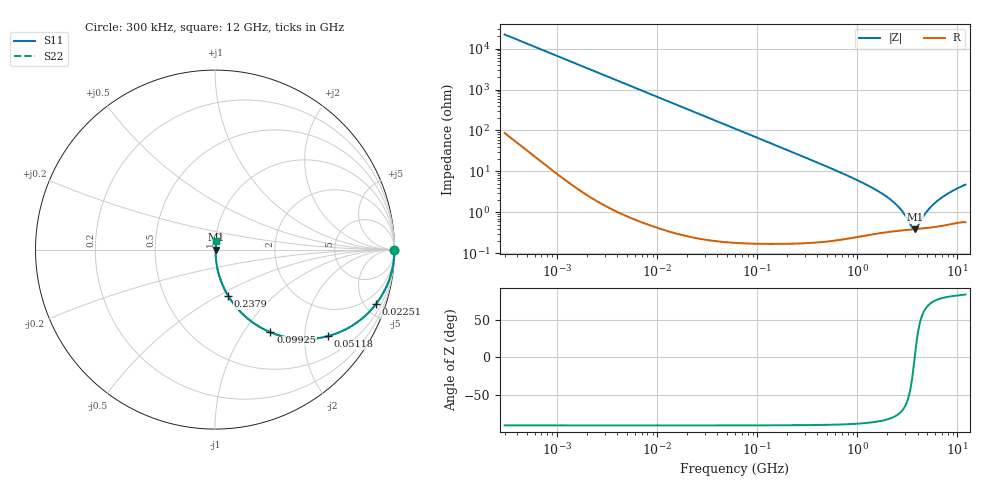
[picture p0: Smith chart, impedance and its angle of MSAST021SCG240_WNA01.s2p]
! MSAST021SCG240_WNA01  S-PARAMETER MODEL  ( Standard Model )
! Model Generated by TAIYO YUDEN Corporation (http://www.ty-top.com)
! Version 1.0
! TAIYO YUDEN Control No. 241126
! Copyright(c) 2024 TAIYO YUDEN CO.,LTD. All Rights Reserved.
! Product Description (link to TY-COMPAS)
! https://ds.yuden.co.jp/TYCOMPAS/or/detail?pn=MSAST021SCG240JWNA01&u=M
! Products Name : Multilayer Ceramic Capacitors
! Characteristics :
!  Capacitance : 24 [pF] , Rated Voltage : 25 [V] , TCC : CG / C0G
!  Case Size : 0.25 x 0.125 / 0.0098 x 0.0049 [mm/inch] , Thickness : 0.125 / 0.0049 [mm/inch]
!  (Conditions: Temperature = 25 [degC] , DC Bias Voltage = 0 [V])
! External Node Assignments :
!  1  o---| |---o  2
! GND o---------o GND
! Frequency Range : 0.3MHz  -  12000MHz  [ 401 STEP ]
# MHZ S RI R 50
! Freq[MHz].  S11 Real  S11 Imag  S21 Real  S21 Imag  S12 Real  S12 Imag  S22 Real  S22 Imag
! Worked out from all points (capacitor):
!   401 points, 300 kHz to 12 GHz, reference 50 ohm
!   read as one part in series: C = 24 pF near 316.3 kHz
!   lowest |Z| = 386 mohm at 3.741 GHz (marker M1)
!   series resonance near 3.741 GHz, so ESL is about 75 pH
!   S11 on the Smith chart (normalised r, x): 300 kHz: open; 22.51 MHz: 1.00, -5.90; 51.18 MHz: 1.00, -2.59; 99.25 MHz: 1.00, -1.34; 237.9 MHz: 1.00, -0.56; 12 GHz: 1.01, +0.09
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0.3  1 -0.00452  3.82e-05 0.00452  3.82e-05 0.00452  1 -0.00452
1.769972  0.9993 -0.0267  0.000734 0.0267  0.000734 0.0267  0.9993 -0.0267
4.84353  0.9947 -0.0726  0.00534 0.0726  0.00534 0.0726  0.9947 -0.0726
10.44266  0.9758 -0.1535  0.0242 0.1535  0.0242 0.1535  0.9758 -0.1535
22.51442  0.8966 -0.304  0.1034 0.304  0.1034 0.304  0.8966 -0.304
33.49947  0.7968 -0.4019  0.2032 0.4019  0.2032 0.4019  0.7968 -0.4019
51.18236  0.6269 -0.4829  0.3731 0.4829  0.3731 0.4829  0.6269 -0.4829
60  0.5502 -0.4967  0.4498 0.4967  0.4498 0.4967  0.5502 -0.4967
99.25425  0.3092 -0.4609  0.6908 0.4609  0.6908 0.4609  0.3092 -0.4609
151.6462  0.1612 -0.3658  0.8388 0.3658  0.8388 0.3658  0.1612 -0.3658
237.9135  0.0729 -0.2569  0.9271 0.2569  0.9271 0.2569  0.0729 -0.2569
353.9943  0.0348 -0.1786  0.9652 0.1786  0.9652 0.1786  0.0348 -0.1786
1105.905  0.00546 -0.0534  0.9945 0.0534  0.9945 0.0534  0.00546 -0.0534
2088.533  0.00376 -0.0211  0.9962 0.0211  0.9962 0.0211  0.00376 -0.0211
2650.866  0.00369 -0.012  0.9963 0.012  0.9963 0.012  0.00369 -0.012
3454.93  0.00379 -0.0027  0.9962 0.0027  0.9962 0.0027  0.00379 -0.0027
3740.715  0.00385 4.84e-07  0.9962 -4.84e-07  0.9962 -4.84e-07  0.00385 4.84e-07
3944.255  0.0039 0.0018  0.9961 -0.0018  0.9961 -0.0018  0.0039 0.0018
5006.236  0.00424 0.00998  0.9958 -0.00998  0.9958 -0.00998  0.00424 0.00998
6026.253  0.00466 0.0167  0.9953 -0.0167  0.9953 -0.0167  0.00466 0.0167
8281.503  0.00586 0.0293  0.9941 -0.0293  0.9941 -0.0293  0.00586 0.0293
12000  0.00786 0.0465  0.9921 -0.0465  0.9921 -0.0465  0.00786 0.0465
